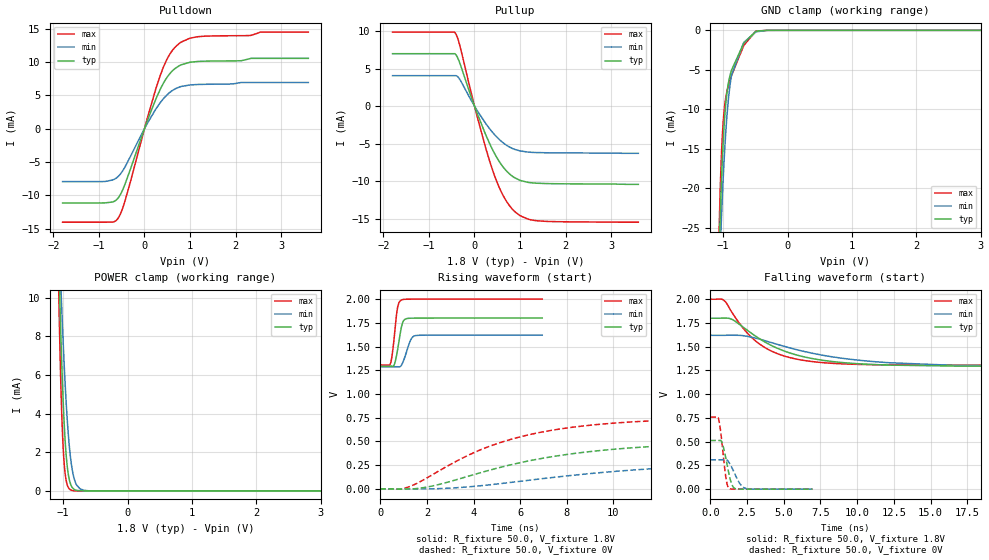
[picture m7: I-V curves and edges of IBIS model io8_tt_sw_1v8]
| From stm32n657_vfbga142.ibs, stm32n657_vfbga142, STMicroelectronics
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[Model]   io8_tt_sw_1v8
Model_type I/O
Polarity   Non-Inverting
Enable   Active-Low
| CAP_THRESHOLD on pad IOTT is "UDTCAPC" :
| Rising=30.0% of vddiov33sw   Falling=70.0% of vddiov33sw
| C_comp min and max val. don't necessarily correlate with the min and max pvt
| but are the smallest and greatest pad capacitance found.
| var   typ   min   max
C_comp   950.41055fF  922.42950fF  979.07055fF
|C_comp_pullup   532.26000fF  524.29000fF  541.88500fF
|C_comp_pulldown   418.15055fF  398.13950fF  437.18555fF
Vinl = 486.0mV
Vinh = 1.4V
Vmeas = 900.0mV   | Reference voltage for timing measurements
Cref  = 50.0pF   | Timing specification test load capacitance value
Rref  = 100.0MOhm   | Timing specification test load resistance value
Vref  = 900.0mV   | Timing specification test load voltage
[Model Spec]
| TIME_THRESHOLD on pin ZIV08SW is "CMOS" :
| Rising=50.0% of vddv08sw   Falling=50.0% of vddv08sw
Vinl 1.07470V 960.70000mV 1.21270V
Vinh 1.54130V 1.38830V 1.70930V
| variable   typ   min   max
[Temperature Range] 25.0 125.0 -40.0
| variable   typ   min   max
[Voltage Range] 1.8V 1.62V 2.0V
| variable   typ   min   max
[POWER Clamp Reference] 1.8V 1.62V 2.0V
| variable   typ   min   max
[GND Clamp Reference] 0V 0V 0V
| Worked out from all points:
|   slope of the pulldown table from 0 to 0.27 V, typ, clamps not added: 56.7 ohm
|   slope of the pullup table from 0 to 0.27 V, typ, clamps not added: 65 ohm
|   GND clamp passes 1 mA (typ) near -0.60 V on its own axis
|   POWER clamp passes 1 mA (typ) near -0.93 V on its own axis
|   rising waveform, R_fixture 50.0, V_fixture 1.8V: 20-80 % time 212ps typ, 275ps min, 183ps max; typ from 1.29 V to 1.8 V
|   falling waveform, R_fixture 50.0, V_fixture 1.8V: 20-80 % time 4.05ns typ, 6.45ns min, 2.82ns max; typ from 1.8 V to 1.29 V
|   rising waveform, R_fixture 50.0, V_fixture 0V: 20-80 % time 6.34ns typ, 9.41ns min, 4.86ns max; typ from 0 V to 0.513 V
|   falling waveform, R_fixture 50.0, V_fixture 0V: 20-80 % time 418ps typ, 596ps min, 330ps max; typ from 0.513 V to 0 V
[POWER Clamp]
-1.8V     154.4mA    107.2mA    224.4mA
-1.07V    12.25mA    13.82mA    10.53mA
-1.05V    9.71mA     11.92mA    7.356mA
-1.03V    7.448mA    10.14mA    4.814mA
-1.01V    5.5mA      8.482mA    2.941mA
-990mV    3.897mA    6.962mA    1.686mA
-970mV    2.647mA    5.596mA    919.9uA
-940mV    1.378mA    3.864mA    349.2uA
-880mV    312.8uA    1.572mA    46.22uA
-790mV    28.91uA    304.1uA    2.176uA
-610mV    235.7nA    8.267uA    28.64nA
3.6V      0A         0A         0A
[GND Clamp]
-1.8V     -1.063A    -785.1mA   -1.154A
-1.06V    -27.67mA   -31.46mA   -24.47mA
-1.05V    -24.83mA   -28.99mA   -21.38mA
-1.03V    -19.89mA   -24.51mA   -16.44mA
-1V       -14.2mA    -18.85mA   -11.67mA
-980mV    -11.44mA   -15.69mA   -9.794mA
-960mV    -9.366mA   -13mA      -8.554mA
-920mV    -6.759mA   -8.872mA   -7.025mA
-870mV    -5.036mA   -5.679mA   -5.739mA
-680mV    -1.634mA   -1.53mA    -1.916mA
-490mV    -108.8uA   -186.8uA   -87.16uA
3.6V      22.62nA    721.2nA    23.49nA
| variable   typ   min   max
[Pullup Reference] 1.8V 1.62V 2.0V
| variable   typ   min   max
[Pulldown Reference] 0V 0V 0V
[Pullup]
-1.8V     6.976mA    4.047mA    9.855mA
-420mV    6.911mA    4.047mA    9.716mA
-330mV    5.842mA    3.611mA    8.232mA
70mV      -1.148mA   -704.5uA   -1.66mA
250mV     -3.883mA   -2.354mA   -5.669mA
420mV     -6.088mA   -3.668mA   -8.932mA
560mV     -7.541mA   -4.541mA   -11.07mA
690mV     -8.567mA   -5.168mA   -12.57mA
850mV     -9.432mA   -5.699mA   -13.86mA
1V        -9.907mA   -5.984mA   -14.61mA
1.56V     -10.33mA   -6.226mA   -15.37mA
3.6V      -10.44mA   -6.3mA     -15.48mA
[Pulldown]
-1.8V     -11.16mA   -7.953mA   -14.05mA
-870mV    -11.15mA   -7.941mA   -14.05mA
-670mV    -10.94mA   -7.622mA   -13.98mA
-570mV    -10.33mA   -7.128mA   -13.35mA
-410mV    -8.002mA   -5.518mA   -10.43mA
70mV      1.323mA    886.5uA    1.768mA
330mV     5.679mA    3.752mA    7.67mA
530mV     8.037mA    5.296mA    10.89mA
760mV     9.437mA    6.239mA    12.79mA
1.18V     10.1mA     6.642mA    13.83mA
2.55V     10.57mA    6.941mA    14.51mA
3.6V      10.57mA    6.941mA    14.51mA
[Ramp]
dV/dt_r 307.61477mV/6.33821ns 185.64768mV/9.1486ns 455.17709mV/4.85595ns
dV/dt_f 304.12359mV/4.04806ns 199.85821mV/6.44848ns 416.78256mV/2.8227ns
R_load = 50.0
| Removed startup time: 0s 0s 0s  .
| Removed end time: 6.95ns.
[Rising Waveform]
R_fixture   = 50.0
V_fixture   = 1.8V
V_fixture_min = 1.62V
V_fixture_max = 2.0V
0s        1.293V     1.287V     1.305V
450ps     1.293V     1.287V     1.327V
600ps     1.308V     1.287V     1.601V
700ps     1.406V     1.287V     1.843V
750ps     1.475V     1.287V     1.922V
900ps     1.697V     1.3V       1.989V
1.05ns    1.785V     1.386V     1.997V
1.3ns     1.798V     1.568V     1.999V
1.5ns     1.799V     1.614V     1.999V
6.95ns    1.8V       1.62V      2V
| Removed startup time: 0s 0s 0s  .
| Removed end time: 74.9ns.
[Falling Waveform]
R_fixture   = 50.0
V_fixture   = 1.8V
V_fixture_min = 1.62V
V_fixture_max = 2.0V
0s        1.8V       1.62V      2V
1ns       1.801V     1.62V      1.978V
1.6ns     1.778V     1.621V     1.832V
2.5ns     1.676V     1.61V      1.648V
4ns       1.526V     1.551V     1.467V
5.6ns     1.425V     1.48V      1.378V
8.2ns     1.346V     1.396V     1.326V
12.2ns    1.306V     1.331V     1.309V
25ns      1.293V     1.29V      1.305V
74.9ns    1.293V     1.287V     1.305V
| Removed startup time: 0s 0s 0s  .
| Removed end time: 74.9ns.
[Rising Waveform]
R_fixture   = 50.0
V_fixture   = 0V
V_fixture_min = 0V
V_fixture_max = 0V
0s        85.85nV    1.055uV    173.6nV
900ps     -2.091mV   -878.1uV   -237.3uV
1.3ns     126.3uV    -1.354mV   28.64mV
2.3ns     34.24mV    1.203mV    158.4mV
4ns       149.6mV    26.42mV    379.9mV
6.1ns     281.4mV    83.06mV    554.4mV
8.7ns     384.7mV    154.3mV    662.9mV
12.1ns    452.8mV    219mV      721.6mV
25ns      508.6mV    296.4mV    757.4mV
74.9ns    512.7mV    309.4mV    758.6mV
| Removed startup time: 0s 0s 0s  .
| Removed end time: 6.95ns.
[Falling Waveform]
R_fixture   = 50.0
V_fixture   = 0V
V_fixture_min = 0V
V_fixture_max = 0V
0s        512.7mV    309.4mV    758.6mV
550ps     512.7mV    309.4mV    748.6mV
800ps     490.5mV    309.4mV    482.2mV
1.05ns    332.4mV    310.1mV    135mV
1.15ns    253.4mV    305.2mV    49.41mV
1.3ns     140.2mV    275mV      6.326mV
1.6ns     15.31mV    184.7mV    858.9uV
2.05ns    730.8uV    50.47mV    375.1uV
2.4ns     381.6uV    8.549mV    250.6uV
6.95ns    38.74uV    60.77uV    21.88uV
